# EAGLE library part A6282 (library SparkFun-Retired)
16-Channel Constant-Current LED Driver Packages: TSSOP-24, 24-pin QFN Last modified: 8/20/10 Unproven! RETIRED! (and wrong category)
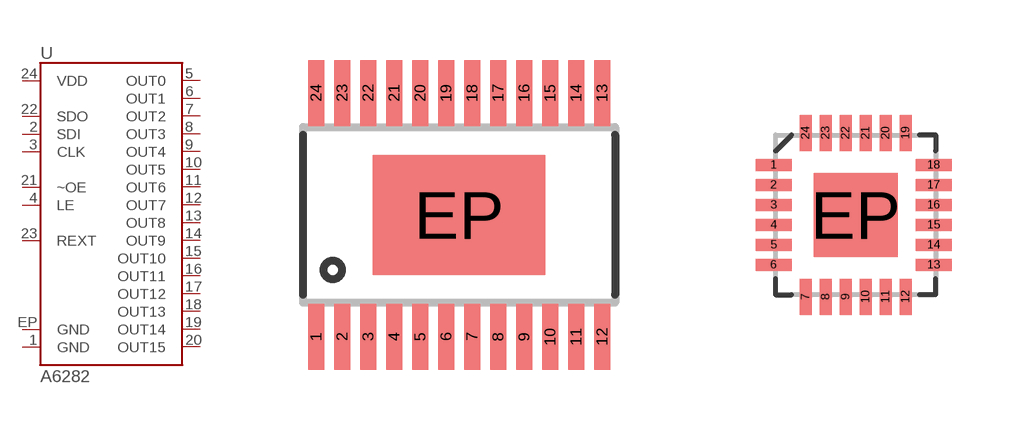
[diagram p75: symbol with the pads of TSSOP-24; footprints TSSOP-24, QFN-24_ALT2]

Designator prefix U

## A6282-LP  [TSSOP-24]
1  GND
2  SDI
3  CLK
4  LE
5  OUT0
6  OUT1
7  OUT2
8  OUT3
9  OUT4
10  OUT5
11  OUT6
12  OUT7
13  OUT8
14  OUT9
15  OUT10
16  OUT11
17  OUT12
18  OUT13
19  OUT14
20  OUT15
21  ~OE
22  SDO
23  REXT
24  VDD
EP  GND

## A6282-ES  [QFN-24_ALT2]
1  SDO
2  REXT
3  VDD
4  GND
5  SDI
6  CLK
7  LE
8  OUT0
9  OUT1
10  OUT2
11  OUT3
12  OUT4
13  OUT5
14  OUT6
15  OUT7
16  OUT8
17  OUT9
18  OUT10
19  OUT11
20  OUT12
21  OUT13
22  OUT14
23  OUT15
24  ~OE
EP  GND

## Footprint TSSOP-24 (pad centres in mm)
24-pin TSSOP with Exposed Thermal Pad Used on: Allegro A6282 16-bit LED driver Last modified: 8/21/10 ***Unproven***
smd 0.4 x 1.65: 1 -3.575,-3.05; 2 -2.925,-3.05; 3 -2.275,-3.05; 4 -1.625,-3.05; 5 -0.975,-3.05; 6 -0.325,-3.05; 7 0.325,-3.05; 8 0.975,-3.05; 9 1.625,-3.05; 10 2.275,-3.05; 11 2.925,-3.05; 12 3.575,-3.05; 13 3.575,3.05; 14 2.925,3.05; 15 2.275,3.05; 16 1.625,3.05; 17 0.975,3.05; 18 0.325,3.05; 19 -0.325,3.05; 20 -0.975,3.05; 21 -1.625,3.05; 22 -2.275,3.05; 23 -2.925,3.05; 24 -3.575,3.05
smd 4.32 x 3: EP 0,0

## Footprint QFN-24_ALT2 (pad centres in mm)
24-pin QFN with Exposed Thermal pad Parts that use this package: A6282 Last modified: 8/20/10 ***UNPROVEN***
smd 0.9 x 0.3: 1 -2.05,1.25; 2 -2.05,0.75; 3 -2.05,0.25; 4 -2.05,-0.25; 5 -2.05,-0.75; 6 -2.05,-1.25; 13 1.95,-1.25; 14 1.95,-0.75; 15 1.95,-0.25; 16 1.95,0.25; 17 1.95,0.75; 18 1.95,1.25
smd 0.3 x 0.9: 7 -1.25,-2.05; 8 -0.75,-2.05; 9 -0.25,-2.05; 10 0.25,-2.05; 11 0.75,-2.05; 12 1.25,-2.05; 19 1.25,2.05; 20 0.75,2.05; 21 0.25,2.05; 22 -0.25,2.05; 23 -0.75,2.05; 24 -1.25,2.05
smd 2.1 x 2.1: EP 0,0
